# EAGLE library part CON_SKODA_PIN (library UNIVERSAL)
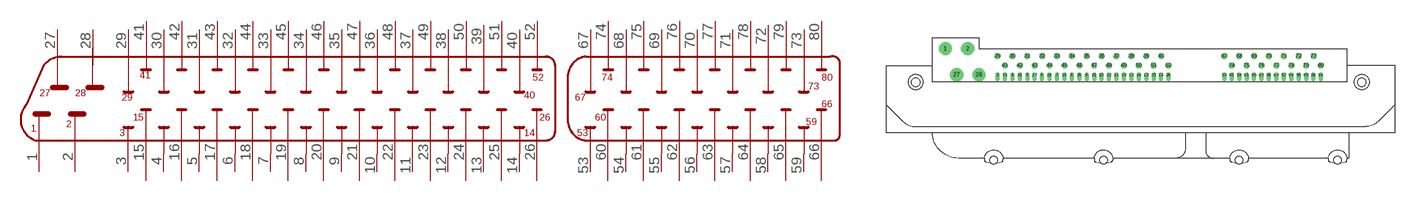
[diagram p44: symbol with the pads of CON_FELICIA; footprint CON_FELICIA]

Designator prefix -

## CON_SKODA_PIN  [CON_FELICIA]
1  P$1
2  P$2
3  P$3
4  P$4
5  P$5
6  P$6
7  P$7
8  P$8
9  P$9
10  P$10
11  P$11
12  P$12
13  P$13
14  P$14
15  P$15
16  P$16
17  P$17
18  P$18
19  P$19
20  P$20
21  P$21
22  P$22
23  P$23
24  P$24
25  P$25
26  P$26
27  P$27
28  P$28
29  P$29
30  P$30
31  P$31
32  P$32
33  P$33
34  P$34
35  P$35
36  P$36
37  P$37
38  P$38
39  P$39
40  P$40
41  P$41
42  P$42
43  P$43
44  P$44
45  P$45
46  P$46
47  P$47
48  P$48
49  P$49
50  P$50
51  P$51
52  P$52
53  P$53
54  P$54
55  P$55
56  P$56
57  P$57
58  P$58
59  P$59
60  P$60
61  P$61
62  P$62
63  P$63
64  P$64
65  P$65
66  P$66
67  P$67
68  P$68
69  P$69
70  P$70
71  P$71
72  P$72
73  P$73
74  P$74
75  P$75
76  P$76
77  P$77
78  P$78
79  P$79
80  P$80

## Footprint CON_FELICIA (pad centres in mm)
drill 0.7 pad 3.81: 1 -14.98,7.49; 2 -8.56,7.49
drill 0.8 pad 1.27 offset: 3 0,0; 4 4.28,0; 5 8.56,0; 6 12.84,0; 7 17.12,0; 8 21.4,0; 9 25.68,0; 10 29.96,0; 11 34.24,0; 12 38.52,0; 13 42.8,0; 14 47.08,0; 15 2.14,0; 16 6.42,0; 17 10.7,0; 18 14.98,0; 19 19.26,0; 20 23.54,0; 21 27.82,0; 22 32.1,0; 23 36.38,0; 24 40.66,0; 25 44.94,0; 26 49.22,0; 53 65.27,0; 54 69.55,0; 55 73.83,0; 56 78.11,0; 57 82.39,0; 58 86.67,0; 59 90.95,0; 60 67.41,0; 61 71.69,0; 62 75.97,0; 63 80.25,0; 64 84.53,0; 65 88.81,0; 66 93.09,0
drill 0.8 pad 3.81: 27 -11.77,0; 28 -5.35,0
drill 0.7 pad 1.676: 29 0,5.35; 30 4.28,5.35; 31 8.56,5.35; 32 12.84,5.35; 33 17.12,5.35; 34 21.4,5.35; 35 25.68,5.35; 36 29.96,5.35; 37 34.24,5.35; 38 38.52,5.35; 39 42.8,5.35; 40 47.08,5.35; 41 2.14,2.675; 42 6.42,2.675; 43 10.7,2.675; 44 14.98,2.675; 45 19.26,2.675; 46 23.54,2.675; 47 27.82,2.675; 48 32.1,2.675; 49 36.38,2.675; 50 40.66,2.675; 51 44.94,2.675; 52 49.22,2.675; 67 65.27,5.35; 68 69.55,5.35; 69 73.83,5.35; 70 78.11,5.35; 71 82.39,5.35; 72 86.67,5.35; 73 90.95,5.35; 74 67.41,2.675; 75 71.69,2.675; 76 75.97,2.675; 77 80.25,2.675; 78 84.53,2.675; 79 88.81,2.675; 80 93.09,2.675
